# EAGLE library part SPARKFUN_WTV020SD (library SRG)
Sparkfun Audio Breakout board for WTV020SD https://www.sparkfun.com/products/11125
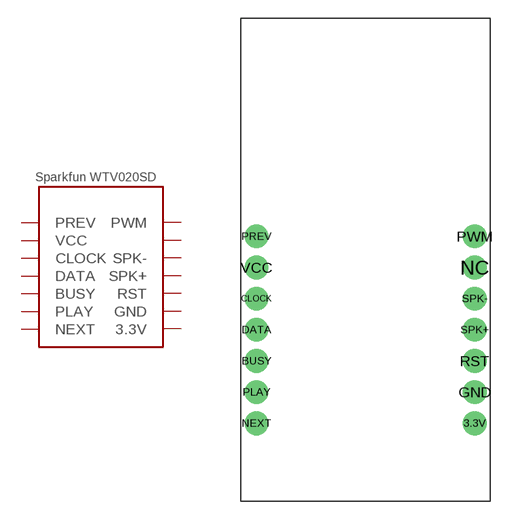
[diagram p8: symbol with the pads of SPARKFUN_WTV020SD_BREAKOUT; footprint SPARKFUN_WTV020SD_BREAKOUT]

Designator prefix -

## SPARKFUN_WTV020SD  [SPARKFUN_WTV020SD_BREAKOUT]
3.3V  3.3V  pwr
BUSY  BUSY  out
CLOCK  CLOCK  in
DATA  DATA
GND  GND  pwr
NC  NC  nc
NEXT  NEXT  in
PLAY  PLAY  in
PREV  PREV  in
PWM  PWM  out
RST  RST  in
SPK+  SPK+  out
SPK-  SPK-  out
VCC  VCC  pwr

## Footprint SPARKFUN_WTV020SD_BREAKOUT (pad centres in mm)
Sparkfun Audio Breakout board for WTV020SD https://www.sparkfun.com/products/11125
drill 1.016 pad 1.93: 3.3V 8.89,-10.16; BUSY -8.89,-5.08; CLOCK -8.89,0; DATA -8.89,-2.54; GND 8.89,-7.62; NC 8.89,2.54; NEXT -8.89,-10.16; PLAY -8.89,-7.62; PREV -8.89,5.08; PWM 8.89,5.08; RST 8.89,-5.08; SPK+ 8.89,-2.54; SPK- 8.89,0; VCC -8.89,2.54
